FUNCTION_BLOCK Example02_shortaxismotion //2x1 flyways w/ 1 xbots - short axis, 6 dof, 6 dof w speed
VAR_INPUT
	Execute : BOOL;
END_VAR
VAR_OUTPUT
	Done : BOOL;
END_VAR
VAR_IN_OUT
	PM_Controller : PMControllerType;	// the planar motor controller to use
END_VAR
VAR
	PMC_XYMotion1 : PMC_XYMotion;
	PMC_ShortAxisMotion1 : PMC_ShortAxisMotion;
	PMC_ShortAxisMotion2 : PMC_ShortAxisMotion;
	PMC_ShortAxisMotion3 : PMC_ShortAxisMotion;
	PMC_6DMotion1 : PMC_6DMotion;
	Pos_array : ARRAY[0..5] OF REAL;
	LongAxisAccVel : ARRAY[0..1] OF REAL;
	ShortAxisVel : ARRAY[0..3] OF REAL;
	PMC_6DMotionVelocity1 : PMC_6DMotionVelocity;
END_VAR

//2x1 flyways w/ 1 xbots - short axis, 6 dof, 6 dof w speed

//move xbot 1 to 120,120
PMC_XYMotion1(Execute := Execute,cmdLB := 1,XbotID := 1,Mode := 0,Type_ := 0,PosX := 0.12,PosY := 0.12,EndVel := 0,MaxVel := 1,MaxAcc := 10,PM_Controller := PM_Controller);

//short axis motion to z = 2 mm
PMC_ShortAxisMotion1(Execute := PMC_XYMotion1.Done,cmdLB := 2,XbotID := 1,Mode := 0,Type_ := 0,PosZ := 0.002,PosRx := 0,PosRy := 0,PosRz := 0,VelZ := 0.1,VelRx := 0.1,VelRy := 0.1,VelRz := 0.1,Cx := 0,Cy := 0,PM_Controller := PM_Controller);

//short axis motion to z = 2 mm, rx = 10mrad, Ry = 10mrad, rz = 80mrad
PMC_ShortAxisMotion2(Execute := PMC_ShortAxisMotion1.Done,cmdLB := 3,XbotID := 1,Mode := 0,Type_ := 0,PosZ := 0.002,PosRx := 0.01,PosRy := 0.01,PosRz := 0.08,VelZ := 0.1,VelRx := 0.1,VelRy := 0.1,VelRz := 0.5,Cx := 0,Cy := 0,PM_Controller := PM_Controller);

//short axis motion to z = 1 mm, rx = 0mrad, Ry = 0mrad, rz = 0mrad
PMC_ShortAxisMotion3(Execute := PMC_ShortAxisMotion2.Done,cmdLB := 4,XbotID := 1,Mode := 0,Type_ := 0,PosZ := 0.001,PosRx := 0.0,PosRy := 0.0,PosRz := 0.0,VelZ := 0.1,VelRx := 0.1,VelRy := 0.1,VelRz := 0.5,Cx := 0.0,Cy := 0.0,PM_Controller := PM_Controller);

//six dof to x=80mm,y=100mm,z=2mm,rx=10mrad,ry=10mrad,rz=80mrad)
PMC_6DMotion1(Execute := PMC_ShortAxisMotion3.Done,cmdLB := 5,XbotID := 1,PosX := 0.08,PosY := 0.1,PosZ := 0.002,PosRx := 0.01,PosRy := 0.01,PosRz := 0.08,PM_Controller := PM_Controller);

//six dof to (120,120,1,0,0,0) w/ user speeds
Pos_array[0] := 0.12;Pos_array[1] := 0.12;Pos_array[2] := 0.001;
LongAxisAccVel[0] := 0.1;LongAxisAccVel[1] := 0.1;
ShortAxisVel[0] := 0.1;ShortAxisVel[1] := 0.1;ShortAxisVel[2] := 0.1;ShortAxisVel[3] := 0.1;
PMC_6DMotionVelocity1(Execute := PMC_6DMotion1.Done,cmdLB := 6,XbotID := 1,TargetPos := Pos_array,LongAxisAccVel := LongAxisAccVel,ShortAxisVel := ShortAxisVel,PM_Controller := PM_Controller);

Done := PMC_6DMotionVelocity1.Done;

END_FUNCTION_BLOCK
